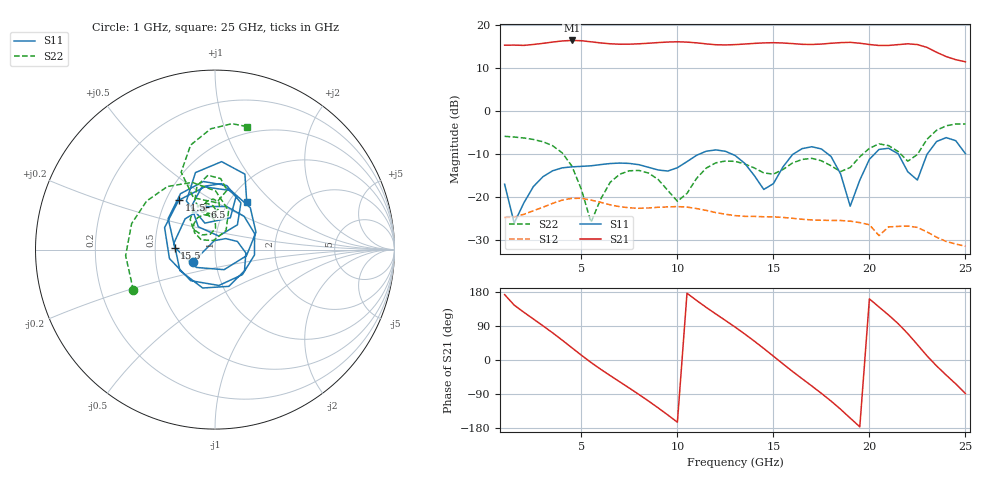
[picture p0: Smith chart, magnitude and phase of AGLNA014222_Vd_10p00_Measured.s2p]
! Filename4Jim: AG19_M068_B_0906_Vd_10p00_CP11_NF.s2p
! Calibration: TFN_AG02, Fixturing for NF
! Notes: Ray
! Row:9, Col:6
! Probes: GSG150
! Prober: TS150
! Date: 2023-12-21 17:27:27
! DC: Vd.V=10.0002, Vd.I=0.0406011, Vg.V=0.372857
! Keysight Technologies,N5245B,MY58421923,A.15.75.19
! AGMDC-PNAX50 Thu Dec 21 17:27:57 2023
# HZ S DB R 50
!freq (Hz)  S11DB  S11A  S21DB  S21A  S12DB  S12A  S22DB  S22A
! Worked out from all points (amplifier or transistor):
!   49 points, 1 GHz to 25 GHz, reference 50 ohm
!   highest |S21| = 16.4 dB at 4.5 GHz (marker M1)
!   |S21| within 3 dB of that: start of sweep to 23.63 GHz
!   unconditionally stable (mu >= 1): start of sweep to end of sweep
!   at 5 GHz: K = 1.04, MAG = 17.1 dB, |S12| = -20.3 dB
!   at 13 GHz: K = 1.43, MAG = 16.0 dB, |S12| = -24.3 dB
!   at 25 GHz: K = 2.35, MAG = 14.9 dB, |S12| = -31.4 dB
!   lowest NFmin = 1.24 dB at 5.5 GHz
!   S11 on the Smith chart (normalised r, x): 1 GHz: 0.77, -0.11; 6.5 GHz: 0.80, +0.41; 11.5 GHz: 0.58, +0.36; 15.5 GHz: 0.63, +0.02; 25 GHz: 1.20, +0.71
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1e9  -17.00 -150.6  15.29 172.5  -24.74 4.8  -5.87 -153.5
1.5e9  -26.03 94.2  15.32 144.8  -24.65 -19.8  -6.04 -176.2
3e9  -15.25 -6.2  15.73 90.1  -22.34 -74.1  -7.13 127.0
4.5e9  -12.97 -107.8  16.40 32.5  -20.29 -140.9  -12.75 70.8
5e9  -12.85 -149.1  16.33 12.6  -20.27 -165.7  -18.21 59.9
6.5e9  -12.19 102.9  15.62 -41.2  -21.79 130.8  -16.55 140.4
8e9  -12.46 21.9  15.62 -91.1  -22.59 78.3  -13.81 108.1
9e9  -13.69 -42.5  15.91 -126.4  -22.35 41.5  -15.91 89.5
1.05e10  -11.74 -168.9  16.01 176.3  -22.32 -21.8  -19.13 132.3
1.15e10  -9.33 126.3  15.60 138.9  -23.07 -64.7  -13.25 129.4
1.3e10  -10.31 49.8  15.43 87.1  -24.29 -123.3  -11.69 99.3
1.4e10  -14.96 -11.0  15.72 50.0  -24.47 -162.6  -13.19 88.5
1.55e10  -12.97 177.1  15.81 -10.3  -24.72 132.4  -13.58 104.9
1.7e10  -8.29 99.7  15.47 -68.6  -25.29 65.9  -10.99 92.0
1.8e10  -10.54 60.9  15.75 -108.2  -25.41 19.5  -12.70 84.0
1.9e10  -22.11 74.6  15.96 -153.2  -25.58 -32.6  -13.11 109.1
2e10  -11.22 118.6  15.46 161.3  -26.41 -87.7  -8.66 105.8
2.1e10  -8.65 84.2  15.24 118.7  -26.91 -141.1  -8.03 85.5
2.2e10  -14.11 64.3  15.62 69.6  -26.71 157.7  -11.66 88.3
2.3e10  -10.06 120.5  14.79 11.0  -28.08 89.7  -6.54 113.6
2.4e10  -6.17 85.7  12.65 -39.8  -30.29 31.3  -3.43 92.0
2.5e10  -9.90 56.5  11.45 -88.5  -31.39 -28.5  -3.00 75.5
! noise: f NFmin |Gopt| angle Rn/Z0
1e+09  1.979  0.2635  -170  0.1278
3.5e+09  1.532  0.3674  -62.59  0.3153
6e+09  1.305  0.2226  -16.22  0.3696
9e+09  1.751  0.007213  -177.4  0.4103
1.15e+10  1.826  0.1511  -56.36  0.3704
1.4e+10  2.185  0.05176  -79.41  0.4765
1.7e+10  2.744  0  90  0.2202
1.95e+10  3.392  0.07938  -103.5  0.7587
2.2e+10  4.753  0.1275  -107.8  1.584
2.5e+10  5.381  0.2893  -91.97  1.264
